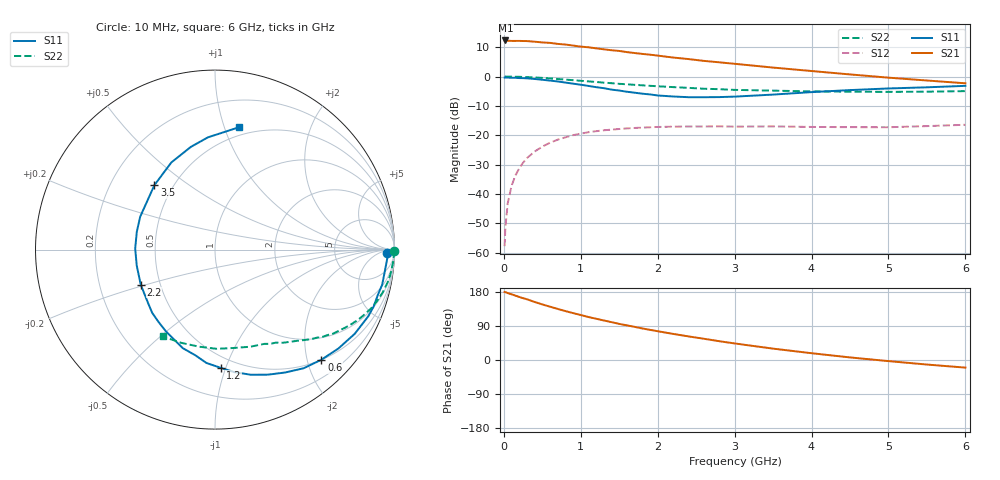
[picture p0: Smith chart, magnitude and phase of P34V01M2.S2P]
! SIEMENS Small Signal Semiconductors
! BFP181
! Si NPN RF Bipolar Junction Transistor in SOT143
! VCE = 4 V  IC = 1.2 mA
! Common Emitter S-Parameters:  March  1996
# GHz  S  MA  R  50
!  f  S11  S21  S12  S22
! GHz  MAG  ANG  MAG  ANG  MAG  ANG  MAG  ANG
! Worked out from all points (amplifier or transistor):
!   36 points, 10 MHz to 6 GHz, reference 50 ohm
!   highest |S21| = 12.3 dB at 20 MHz (marker M1)
!   |S21| within 3 dB of that: start of sweep to 1.296 GHz
!   unconditionally stable (mu >= 1): 2.934 GHz to end of sweep
!   at 250 MHz: K = 0.09, MSG = 20.7 dB, |S12| = -29.3 dB
!   at 1.4 GHz: K = 0.53, MSG = 13.5 dB, |S12| = -18.1 dB
!   at 6 GHz: K = 1.23, MAG = 4.2 dB, |S12| = -16.4 dB
!   S11 on the Smith chart (normalised r, x): 10 MHz: 40, -16; 600 MHz: 0.50, -2.26; 1.2 GHz: 0.41, -0.96; 2.2 GHz: 0.39, -0.19; 3.5 GHz: 0.39, +0.37; 6 GHz: 0.43, +1.12
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0.01  0.9582 -1.0  4.077 179.5  0.0013 92.2  0.9985 -0.4
0.02  0.9639 -1.7  4.109 179.2  0.0027 88.9  0.9981 -0.7
0.05  0.9592 -3.8  4.075 176.6  0.0069 91.0  0.9965 -1.9
0.1  0.9532 -7.9  4.036 173.3  0.0138 83.4  0.9959 -3.6
0.15  0.9517 -11.9  4.036 169.9  0.0207 81.7  0.9914 -5.5
0.3  0.9313 -23.5  4.011 160.3  0.0409 75.2  0.9786 -10.8
0.4  0.9089 -31.1  3.914 153.2  0.0529 70.0  0.9648 -14.2
0.6  0.853 -46.0  3.738 140.7  0.0748 60.5  0.9297 -20.6
0.8  0.7888 -60.2  3.501 129.1  0.0924 52.2  0.8882 -26.1
1.1  0.6919 -80.9  3.144 113.4  0.113 41.9  0.8262 -33.1
1.2  0.6592 -87.3  3.017 108.9  0.1175 38.6  0.8079 -35.4
1.5  0.5776 -108.1  2.723 95.3  0.128 31.0  0.7515 -40.7
1.8  0.5105 -128.3  2.427 83.2  0.1353 24.8  0.7087 -45.3
2.2  0.4576 -154.7  2.104 68.9  0.1403 18.0  0.6608 -51.1
2.4  0.445 -168.6  1.982 62.3  0.1414 15.1  0.6417 -54.0
2.8  0.4468 167.1  1.746 49.6  0.142 10.8  0.6091 -59.5
3  0.4553 156.3  1.647 43.7  0.1406 9.0  0.5927 -62.4
3.5  0.493 133.2  1.42 30.0  0.1417 5.8  0.5758 -70.0
4  0.5431 116.6  1.241 17.9  0.1388 3.9  0.5583 -79.0
4.5  0.588 103.2  1.086 6.8  0.1376 2.2  0.5527 -89.1
5.5  0.6556 85.8  0.856 -12.0  0.1434 4.4  0.5527 -110.1
6  0.694 79.0  0.767 -20.1  0.1512 4.2  0.5646 -121.0
